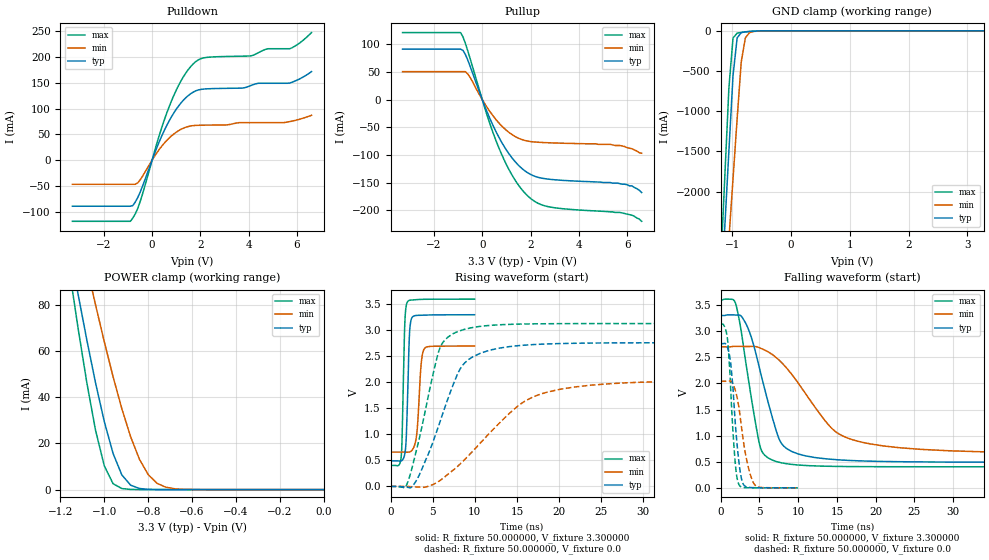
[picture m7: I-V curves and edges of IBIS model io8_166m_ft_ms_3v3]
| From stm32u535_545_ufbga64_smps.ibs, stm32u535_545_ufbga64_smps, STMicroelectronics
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|   Model io8_166m_ft_ms_3v3
[Model]  io8_166m_ft_ms_3v3
Model_type I/O
Polarity   Non-Inverting
Enable   Active-Low
Vinl =   0.990000V
Vinh =   2.310000V
Vmeas =  1.650000V
Cref =   50.000000pF
Rref =   100.000000M
Vref =   0.0V
C_comp   3.517200pF   3.489400pF   3.557800pF
[Temperature Range]   25.000000   0.140000k   -40.000000
[Pullup Reference]   3.300000V   2.700000V   3.600000V
[Pulldown Reference]   0.0V   0.0V   0.0V
[POWER Clamp Reference]   3.300000V   2.700000V   3.600000V
[GND Clamp Reference]   0.0V   0.0V   0.0V
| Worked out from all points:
|   slope of the pulldown table from 0 to 0.495 V, typ, clamps not added: 8.73 ohm
|   slope of the pullup table from 0 to 0.495 V, typ, clamps not added: 9.64 ohm
|   GND clamp passes 1 mA (typ) near -0.50 V on its own axis
|   POWER clamp passes 1 mA (typ) near -0.85 V on its own axis
|   rising waveform, R_fixture 50.000000, V_fixture 3.300000: 20-80 % time 306ps typ, 454ps min, 272ps max; typ from 0.49 V to 3.3 V
|   rising waveform, R_fixture 50.000000, V_fixture 0.0: 20-80 % time 3.81ns typ, 7.78ns min, 2.6ns max; typ from 0 V to 2.76 V
|   falling waveform, R_fixture 50.000000, V_fixture 3.300000: 20-80 % time 3.01ns typ, 6.39ns min, 2.05ns max; typ from 3.3 V to 0.49 V
|   falling waveform, R_fixture 50.000000, V_fixture 0.0: 20-80 % time 901ps typ, 1.3ns min, 737ps max; typ from 2.76 V to 0 V
[Pulldown]
|Voltage   I(typ)   I(min)   I(max)
-3.3V     -89.72mA   -47.06mA   -119mA
-900mV    -89.72mA   -47.06mA   -119mA
-500mV    -62.92mA   -38.71mA   -81.44mA
300mV     36.2mA     21.01mA    48.7mA
800mV     84.07mA    46.96mA    114.8mA
1.3V      116.7mA    62.09mA    162.4mA
1.8V      134.4mA    67.39mA    191.2mA
2.3V      138.6mA    67.98mA    199.8mA
4.1V      145.2mA    72.79mA    202.7mA
4.8V      149.4mA    72.79mA    216.5mA
5.7V      149.8mA    74.8mA     216.5mA
6.6V      172mA      87.1mA     247.9mA
[Pullup]
|Voltage   I(typ)   I(min)   I(max)
-3.3V     91.09mA    50.39mA    121mA
-900mV    91.09mA    50.39mA    121mA
-800mV    88.97mA    50.39mA    113.5mA
-600mV    71.54mA    46.26mA    88.13mA
200mV     -22.26mA   -14.13mA   -28.39mA
700mV     -69mA      -42.82mA   -88.5mA
1.3V      -109.1mA   -65.19mA   -141.4mA
2V        -135.3mA   -75.91mA   -178.7mA
2.9V      -144.6mA   -78.33mA   -194.9mA
5.3V      -150mA     -81mA      -203mA
6.2V      -156mA     -89mA      -209mA
6.6V      -168mA     -97mA      -220mA
[GND_clamp]
|Voltage   I(typ)   I(min)   I(max)
-3.3V     -9.098A    -9.372A    -9.671A
-1.2V     -3.386A    -4.091A    -2.933A
-1.13V    -2.437A    -3.34A     -1.815A
-1.06V    -1.49A     -2.588A    -705.6mA
-990mV    -555.7mA   -1.839A    -89.03mA
-920mV    -88.12mA   -1.093A    -28.78mA
-850mV    -22.35mA   -387.4mA   -19.84mA
-780mV    -12.12mA   -88.01mA   -13.88mA
-710mV    -7.71mA    -22.52mA   -8.846mA
-640mV    -4.545mA   -7.864mA   -4.87mA
-360mV    -31.12uA   -173.5uA   -8.497uA
3.28V     0A         14.15nA    -7.901nA
[POWER_clamp]
|Voltage   I(typ)   I(min)   I(max)
-3.28V    1.355A     1.167A     1.664A
-1.16V    105.7mA    131.6mA    95.69mA
-1.12V    84.97mA    114mA      70.27mA
-1.08V    65.05mA    96.83mA    46.54mA
-1.04V    46.34mA    80.15mA    25.76mA
-1V       29.51mA    64.13mA    10.3mA
-960mV    15.69mA    48.99mA    2.571mA
-920mV    6.373mA    35.1mA     455.6uA
-840mV    490.7uA    13.24mA    11.36uA
-760mV    27.33uA    2.767mA    278.3nA
-640mV    347.6nA    134.1uA    16.77nA
0V        0A         19.95nA    0A
[Ramp]
| variable   typ   min   max
dV/dt_r  1.65714/3.80352n   1.22436/7.77639n   1.87854/2.59311n
dV/dt_f  1.68605/3.01059n   1.22255/6.37587n   1.91789/2.04514n
R_load = 50.000000
[Rising Waveform]
R_fixture= 50.000000
V_fixture= 3.300000
V_fixture_min= 2.700000
V_fixture_max= 3.600000
|time   V(typ)   V(min)   V(max)
0s        489.9mV    659.8mV    403.5mV
1.261ns   490.9mV    659.8mV    572.4mV
1.682ns   622.4mV    659.5mV    3.098V
1.982ns   1.515V     658.3mV    3.541V
2.242ns   2.914V     661.9mV    3.577V
2.583ns   3.254V     702.4mV    3.584V
3.103ns   3.287V     999.6mV    3.591V
3.604ns   3.29V      2.298V     3.595V
3.964ns   3.292V     2.636V     3.597V
9.97ns    3.3V       2.7V       3.6V
[Rising Waveform]
R_fixture= 50.000000
V_fixture= 0.0
V_fixture_min= 0.0
V_fixture_max= 0.0
|time   V(typ)   V(min)   V(max)
0s        5.268uV    5.723uV    3.567uV
1.802ns   -13.17mV   184.6uV    -5.448mV
3.003ns   97.32mV    -9.834mV   653.6mV
5.766ns   1.195V     103.3mV    2.619V
6.727ns   1.648V     222.4mV    2.858V
8.408ns   2.295V     454.7mV    3.001V
10.57ns   2.553V     818.9mV    3.075V
15.26ns   2.707V     1.562V     3.12V
20.18ns   2.746V     1.869V     3.129V
59.82ns   2.762V     2.041V     3.131V
[Falling Waveform]
R_fixture= 50.000000
V_fixture= 3.300000
V_fixture_min= 2.700000
V_fixture_max= 3.600000
|time   V(typ)   V(min)   V(max)
0s        3.3V       2.7V       3.6V
1.922ns   3.309V     2.709V     3.533V
3.363ns   3.111V     2.707V     2.283V
5.165ns   2.193V     2.672V     751.7mV
7.087ns   1.132V     2.503V     508.5mV
7.928ns   834.2mV    2.389V     476.4mV
9.249ns   691.3mV    2.158V     448.2mV
14.29ns   547mV      1.146V     412.3mV
18.02ns   516.5mV    881.5mV    406.7mV
59.82ns   489.9mV    659.8mV    403.5mV
[Falling Waveform]
R_fixture= 50.000000
V_fixture= 0.0
V_fixture_min= 0.0
V_fixture_max= 0.0
|time   V(typ)   V(min)   V(max)
0s        2.762V     2.041V     3.131V
800.8ps   2.713V     2.041V     2.924V
1.201ns   2.483V     2.046V     2.168V
1.562ns   1.956V     1.994V     1.131V
1.822ns   1.368V     1.9V       578.4mV
2.342ns   508.6mV    1.546V     67.63mV
2.943ns   63.98mV    880.7mV    6.298mV
3.584ns   10.16mV    383.7mV    2.303mV
4.364ns   3.346mV    64.62mV    1.198mV
9.97ns    5.268uV    5.723uV    3.567uV
